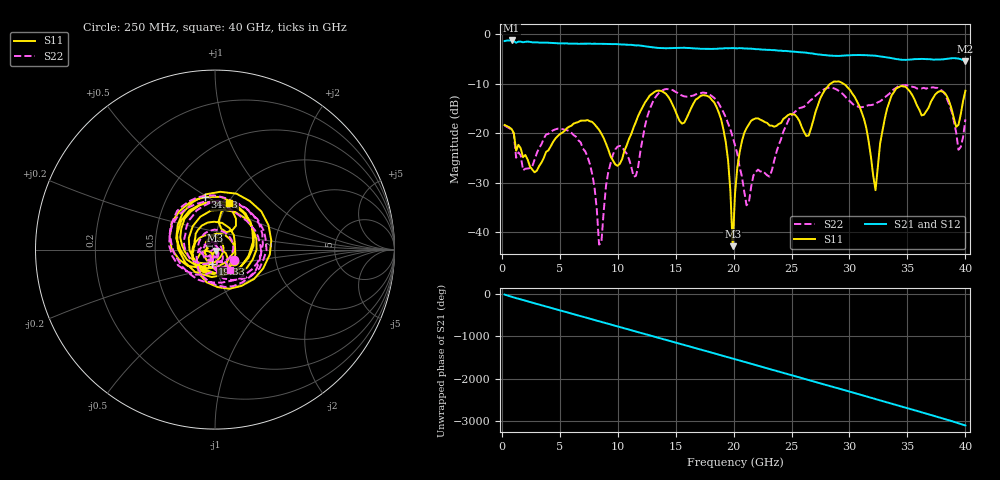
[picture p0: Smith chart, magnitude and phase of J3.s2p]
!Agilent Technologies,E8364B,MY43040528,A.07.50.67
!Agilent E8364B: A.07.50.67
!Date: Thursday, May 22, 2025 22:51:44
!Correction: S11(Full 2 Port(1,2))
!S21(Full 2 Port(1,2))
!S12(Full 2 Port(1,2))
!S22(Full 2 Port(1,2))
!S2P File: Measurements: S11, S21, S12, S22:
# Hz S  dB  R 50
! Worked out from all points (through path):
!   201 points, 250 MHz to 40 GHz, reference 50 ohm
!   highest |S21| = -1.22 dB at 846.2 MHz (marker M1); lowest = -5.5 dB at 40 GHz (marker M2)
!   group delay of S21, straight-line fit = 214 ps
!   lowest |S11| = -42.9 dB at 19.93 GHz (marker M3), VSWR 1.01, Z = 50.3 - j0.656 ohm
!   |S11| at or under -10 dB: start of sweep to 28.35 GHz; 29.49 GHz to end of sweep
!   |S22| runs from -42.5 to -10.3 dB; largest |S21 - S12| = 0.0062
!   S11 on the Smith chart (normalised r, x): 250 MHz: 1.22, -0.16; 19.33 GHz: 0.96, -0.15; 34.63 GHz: 0.76, +0.49; 40 GHz: 1.01, +0.56
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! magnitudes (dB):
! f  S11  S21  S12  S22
! 250 MHz  -18.3  -1.3  -1.3  -18.5
! 846.2 MHz  -19.1  -1.2  -1.2  -19.3
! 2.834 GHz  -27.9  -1.6  -1.6  -25.4
! 7.008 GHz  -17.4  -1.9  -1.9  -23.1
! 8.001 GHz  -18.2  -1.9  -1.9  -30.8
! 8.399 GHz  -19.3  -1.9  -1.9  -42.5
! 9.591 GHz  -25.5  -2.0  -1.9  -24.3
! 11.58 GHz  -17.7  -2.2  -2.2  -28.6
! 13.57 GHz  -11.4  -2.7  -2.7  -11.8
! 15.55 GHz  -18.0  -2.7  -2.7  -12.4
! 17.94 GHz  -12.7  -2.9  -2.9  -12.2
! 19.33 GHz  -21.8  -2.8  -2.8  -16.8
! 19.93 GHz  -42.9  -2.8  -2.8  -20.8
! 20.12 GHz  -32.3  -2.8  -2.8  -22.4
! 21.12 GHz  -19.0  -2.9  -2.9  -34.6
! 26.88 GHz  -17.4  -3.9  -3.9  -13.0
! 30.06 GHz  -11.3  -4.2  -4.2  -13.6
! 32.25 GHz  -31.5  -4.3  -4.3  -14.0
! 33.44 GHz  -13.7  -4.7  -4.7  -12.0
! 34.63 GHz  -10.5  -5.1  -5.1  -10.3
! 39.2 GHz  -18.7  -4.8  -4.8  -19.9
! 40 GHz  -11.4  -5.5  -5.4  -17.2
